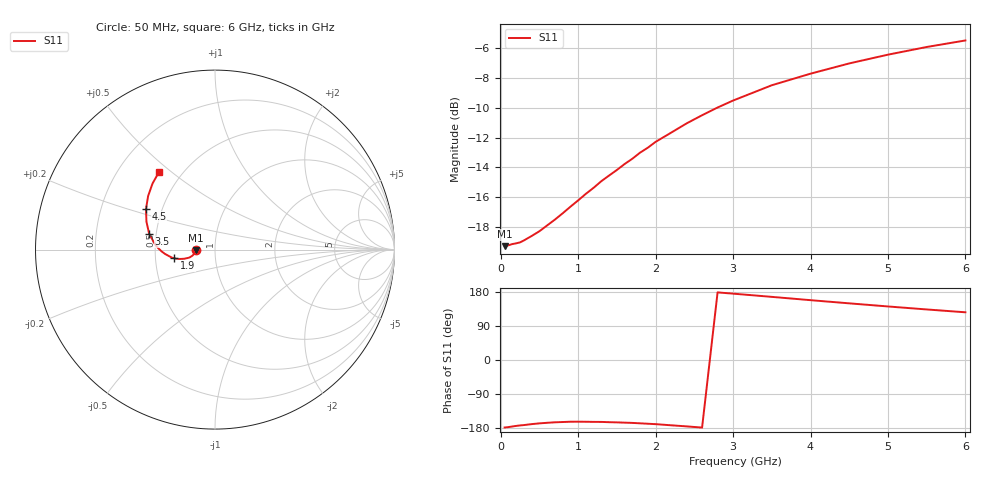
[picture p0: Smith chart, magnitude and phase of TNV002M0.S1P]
! SIEMENS Discrete & RF Semiconductors
! BAS70-07W
! Si Schottky Diode in SOT343
! IF = 2 mA
! S-Parameters:  February  1997
# GHz  S  MA  R  50
!  f  S11
! GHz  MAG  ANG
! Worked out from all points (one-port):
!   34 points, 50 MHz to 6 GHz, reference 50 ohm
!   lowest |S11| = -19.3 dB at 50 MHz (marker M1), VSWR 1.24, Z = 40.2 - j0.278 ohm
!   |S11| at or under -10 dB: start of sweep to 2.789 GHz
!   S11 on the Smith chart (normalised r, x): 50 MHz: 0.80, -0.01; 1.9 GHz: 0.63, -0.06; 3.5 GHz: 0.46, +0.09; 4.5 GHz: 0.41, +0.23; 6 GHz: 0.38, +0.45
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0.05  0.1086 -178.2
0.15  0.1104 -175.4
0.25  0.1118 -172.6
0.3  0.1135 -171.7
0.5  0.1219 -167.2
0.7  0.1334 -164.4
0.8  0.14 -163.7
0.9  0.1473 -162.9
1  0.1547 -162.8
1.1  0.1628 -163.0
1.2  0.1706 -163.3
1.3  0.1796 -163.4
1.5  0.1958 -164.6
1.6  0.205 -165.3
1.7  0.2135 -166.0
1.8  0.2239 -167.1
1.9  0.2326 -168.2
2  0.2433 -169.3
2.4  0.2806 -175.2
2.6  0.2989 -178.3
2.8  0.3173 178.4
3  0.3348 175.1
3.5  0.3769 166.6
4  0.4122 157.9
4.5  0.4462 149.5
5  0.4775 141.3
5.5  0.5066 133.4
6  0.5329 125.9
